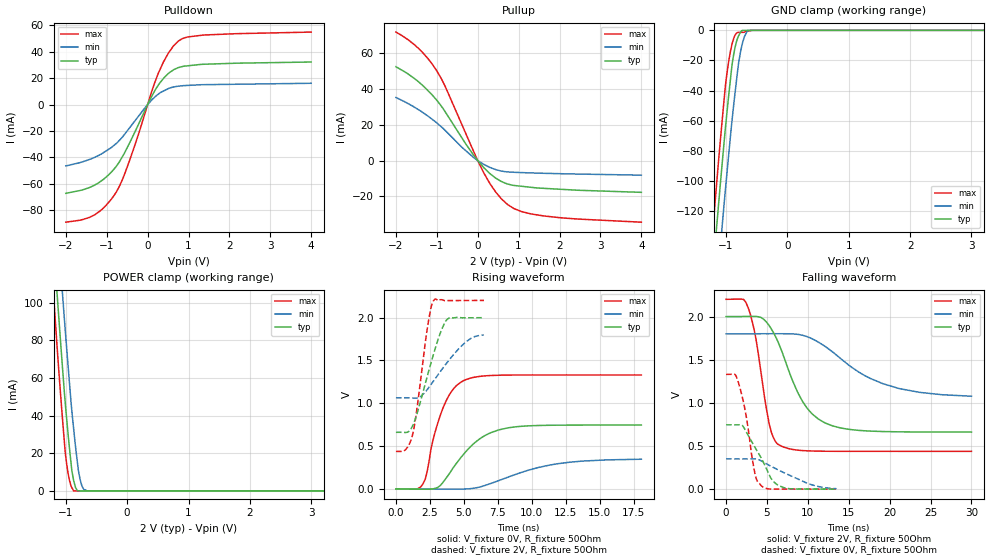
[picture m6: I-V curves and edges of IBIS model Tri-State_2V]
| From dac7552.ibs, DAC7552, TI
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|   Model   - Tristate_2V
[Model]   Tri-State_2V
Model_type   3-state
Polarity   Non-Inverting
Enable   Active-High
Vmeas = 1
Vref = 1
Cref = 15pF
Rref = 50
|   typ   min   max
|   (nom PVT)   (Fast PVT)   (slow PVT)
|Average
C_comp   2.726e-12   2.248e-12   3.219e-12
|ON state : BUFFER OUTPUT TURNED HIGH
|C_comp   4.613e-12   3.668e-12   5.586e-12
|OFF state: BUFFER in HIGH IMPEDANCE for IOs and 3-state,
|This is BUFFER in LOW state for OUTPUT only type
|C_comp   8.395e-13   8.287e-13   8.527e-13
| Where   nom  PVT is  Nominal Process, 2.0V, 25C
|   Fast PVT is Strong Process, 2.2V, -40C
|   Slow PVT is Weak Process, 1.8V, 105C
[Voltage Range]   2   1.8   2.2
|Ambient Temperature   25   105   -40
|Junction Temperature
[Temperature Range]   25   105   -40
[Pullup Reference]   2   1.8   2.2
[Pulldown Reference]   0   0   0
[Power Clamp Reference]   2   1.8   2.2
[GND Clamp Reference]   0   0   0
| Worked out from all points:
|   slope of the pulldown table from 0 to 0.3 V, typ, clamps not added: 18.2 ohm
|   slope of the pullup table from 0 to 0.3 V, typ, clamps not added: 41 ohm
|   GND clamp passes 1 mA (typ) near -0.76 V on its own axis
|   POWER clamp passes 1 mA (typ) near -0.83 V on its own axis
|   falling waveform, V_fixture 2V, R_fixture 50Ohm: 20-80 % time 3.77ns typ, 7.11ns min, 1.78ns max; typ from 2 V to 0.661 V
|   rising waveform, V_fixture 0V, R_fixture 50Ohm: 20-80 % time 2.48ns typ, 4.21ns min, 1.44ns max; typ from 0 V to 0.745 V
|   rising waveform, V_fixture 2V, R_fixture 50Ohm: 20-80 % time 1.43ns typ, 2.17ns min, 874ps max; typ from 0.661 V to 2 V
|   falling waveform, V_fixture 0V, R_fixture 50Ohm: 20-80 % time 2.5ns typ, 4.6ns min, 1.37ns max; typ from 0.745 V to 0 V
[Pulldown]
|   Voltage   I(typ)   I(min)   I(max)
-2V       -67.17mA   -46.44mA   -89mA
-1.292V   -60.85mA   -39.88mA   -83.36mA
-1.023V   -55.08mA   -35.26mA   -76.52mA
-768mV    -46.82mA   -29.47mA   -66.33mA
-618.4mV  -39.53mA   -24.71mA   -56.97mA
-442.4mV  -29.16mA   -17.64mA   -42.43mA
60mV      3.926mA    2.025mA    5.968mA
261.6mV   14.76mA    7.894mA    23.64mA
508mV     23.55mA    12.08mA    38.98mA
752.2mV   28mA       13.95mA    48.07mA
1.37V     30.52mA    15.07mA    52.65mA
4V        32.21mA    16.13mA    54.87mA
[GND Clamp]
|   Voltage   I(typ)   I(min)   I(max)
-2V       -561.4mA   -593.5mA   -542.2mA
-1.252V   -178.4mA   -218.9mA   -150.5mA
-1.199V   -152.6mA   -193.4mA   -124.3mA
-1.164V   -135.6mA   -176.8mA   -106.9mA
-1.078V   -95.31mA   -136.7mA   -66.5mA
-1.036V   -76.01mA   -117.3mA   -47.83mA
-928.6mV  -32.62mA   -70.5mA    -14.01mA
-878mV    -16.6mA    -50.56mA   -5.694mA
-814.2mV  -5.499mA   -27.84mA   -1.432mA
-729.2mV  0A         -7.918mA   -1.335mA
-644.6mV  0A         0A         -522.9uA
4V        0A         0A         0A
[Pullup]
|   Voltage   I(typ)   I(min)   I(max)
-2V       52.34mA    35.19mA    71.68mA
-1.454V   44.08mA    28.47mA    62.71mA
-1.223V   39.17mA    24.93mA    57.07mA
-1.012V   33.97mA    21.23mA    50.46mA
-787.8mV  26.92mA    16.59mA    40.99mA
-136mV    4.147mA    2.385mA    6.931mA
151.6mV   -4.04mA    -2.158mA   -7.031mA
439.8mV   -9.809mA   -5.05mA    -17.58mA
730.2mV   -13.07mA   -6.337mA   -24.52mA
1.067V    -14.33mA   -6.713mA   -28.43mA
1.599V    -15.47mA   -7.097mA   -30.86mA
4V        -17.73mA   -8.14mA    -34.38mA
[POWER Clamp]
|   Voltage   I(typ)   I(min)   I(max)
-2V       538.6mA    569mA      521.8mA
-1.22V    141.8mA    180.9mA    114.4mA
-1.173V   119.5mA    158.7mA    91.43mA
-1.138V   103.1mA    142.6mA    74.89mA
-1.054V   65.61mA    104.9mA    38.39mA
-1.008V   46.43mA    84.96mA    20.12mA
-963.8mV  30.53mA    66.91mA    9.558mA
-902mV    10.99mA    42.79mA    1.743mA
-872mV    5.502mA    33.06mA    0A
-768.8mV  0A         6.406mA    0A
-662mV    0A         69.96uA    0A
4V        0A         0A         0A
[Ramp]
R_load = 50
|   typ   min   max
dV/dt_r   0.44725/2.47462e-09   0.210001/4.27427e-09   0.797986/1.43335e-09
dV/dt_f   0.803364/3.75853e-09   0.43395/7.10954e-09   1.05729/1.77426e-09
[Falling Waveform]
V_fixture = 2V
V_fixture_min = 1.8V
V_fixture_max = 2.2V
R_fixture = 50Ohm
C_fixture = 0F
|   Time   V(typ)   V(min)   V(max)
0s        2V         1.8V       2.2V
2.15ns    2.002V     1.8V       2.198V
2.725ns   2.002V     1.8V       2.098V
3.625ns   2.002V     1.8V       1.756V
5.275ns   1.895V     1.801V     756.7mV
6.35ns    1.707V     1.801V     519.9mV
9.3ns     1.025V     1.785V     447.2mV
12.17ns   764mV      1.65V      439mV
19.2ns    667.3mV    1.221V     437.9mV
30ns      661.1mV    1.077V     437.9mV
[Rising Waveform]
V_fixture = 0V
V_fixture_min = 0V
V_fixture_max = 0V
R_fixture = 50Ohm
C_fixture = 0F
|   Time   V(typ)   V(min)   V(max)
0s        612pV      873.9pV    471pV
1.95ns    -2.463mV   -843.4uV   49.69mV
2.85ns    5.466mV    -1.571mV   645.5mV
3.45ns    74.18mV    -1.78mV    939.2mV
4.225ns   250.6mV    -2.064mV   1.167V
4.975ns   404.4mV    -1.326mV   1.264V
6.5ns     618.7mV    37.84mV    1.319V
8.3ns     714.3mV    141mV      1.329V
11.92ns   744.1mV    294.7mV    1.33V
18.05ns   745.4mV    346.7mV    1.33V
[Rising Waveform]
V_fixture = 2V
V_fixture_min = 1.8V
V_fixture_max = 2.2V
R_fixture = 50Ohm
C_fixture = 0F
|   Time   V(typ)   V(min)   V(max)
0s        661mV      1.064V     437.9mV
700ps     658.7mV    1.064V     457.6mV
1.225ns   735.7mV    1.061V     633.5mV
1.525ns   865mV      1.061V     914.1mV
2.325ns   1.325V     1.164V     1.889V
2.75ns    1.564V     1.256V     2.192V
3.35ns    1.854V     1.388V     2.209V
3.8ns     1.984V     1.482V     2.198V
5.45ns    1.998V     1.751V     2.2V
6.475ns   1.999V     1.797V     2.2V
[Falling Waveform]
|Gnd
V_fixture = 0V
V_fixture_min = 0V
V_fixture_max = 0V
R_fixture = 50Ohm
C_fixture = 0F
|   Time   V(typ)   V(min)   V(max)
0s        745.4mV    350mV      1.33V
1.075ns   745.4mV    350mV      1.33V
1.5ns     745.2mV    350mV      1.239V
2.375ns   680.3mV    350mV      891mV
3.575ns   478.1mV    350.7mV    160.5mV
4.275ns   364mV      328mV      42.16mV
5.525ns   121.3mV    263.4mV    -504.3uV
6.525ns   36.65mV    215.3mV    576.6uV
10.35ns   481.5uV    53.61mV    26.41uV
13.5ns    120uV      4.449mV    1.734uV
